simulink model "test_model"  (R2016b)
settings: Solver=VariableStepAuto  StartTime=0.0  StopTime=runtime  RelTol=1e-3
InitFcn:
  | clear mex
  | delete test_model_sfun.mexw64
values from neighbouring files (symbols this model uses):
  delta_T = 4 * [ 0,  0,  2.351e-4 ]    [modelParameters.m]
  Delta_T = cell(1,4)    [modelParameters.m]
  F_D = 1*randn(3,1)    [modelParameters.m]
  g = 9.81    [modelParameters.m]    (also in analyzeIMU_data.m = 9.8; getMomentOfInertia.m = 9.80665)
  Gamma_H = cell(1,4)    [modelParameters.m]
  have_motor_transient = 1    [modelParameters.m]
  height_controlled_o = (((Rm*If        + (((omega0_o * 2 * Rm * Kv * Kq      * Kd + 1)^2) - 1)/(4* Rm*Kv^2*Kq      * Kd))/Vb)*(Pmax - Pmin) + Pmin)    [modelParameters.m]
  i_0 = cell(1,4)    [modelParameters.m]
  If = 0.3836    [modelParameters.m]    (also in thrustDragConstantCalculations.m = [If0; If1; If2; If3]; Kd_error.m = I_0 * sign(rotor_speed_0) + I_1 * rotor_speed_0 + I_2 * roto)
  J = diag([ 0.0130 0.0140 0.0285 ])    [modelParameters.m]    (also in J_calc_bifilar.m = (16*pi^2*L./(m*g.*D.^2))\(t./n).^2)
  J_L = m_L/12*diag([y_L^2+z_L^2,x_L^2+z_L^2,x_L^2+y_L^2])    [modelParameters.m]
  J_r = cell(1,4)    [modelParameters.m]
  Jreq = 4.2012e-05    [modelParameters.m]
  Jxx = 0.0130    (= 0.013)    [modelParameters.m]
  Jyy = 0.0140    (= 0.014)    [modelParameters.m]
  Jzz = 0.0285    [modelParameters.m]
  K_d = cell(1,4)    [modelParameters.m]
  K_E = cell(1,4)    [modelParameters.m]
  K_H = cell(1,4)    [modelParameters.m]
  K_Q = cell(1,4)    [modelParameters.m]
  K_T = cell(1,4)    [modelParameters.m]
  K_V = cell(1,4)    [modelParameters.m]
  Kd = 1.4852e-07    [modelParameters.m]    (also in calcDragConstant.m = ((A'*A)^-1)*A'*b; thrustDragConstantCalculations.m = calcDragConstant(data, Pmin, Pmax, Rm, Kv, Kq, If); Kd_error.m = 1.0317e-07)
  Kh = 3.4574e-04    (= 0.00034574)    [modelParameters.m]
  Ki_mahony = 0.001    [modelParameters.m]
  Kp_mahony = 0.4    [modelParameters.m]
  Kq = 96.3422    [modelParameters.m]    (also in thrustDragConstantCalculations.m; Kd_error.m)
  Kt = 1.2007e-05    [modelParameters.m]    (also in calcThrustConstant.m = ((A'*A)^(-1))*(A'*T); thrustDragConstantCalculations.m = calcThrustConstant(data))
  Kv = 96.3422    [modelParameters.m]    (also in thrustDragConstantCalculations.m; Kd_error.m)
  m = 1.216    [modelParameters.m]
  m_L = 0    [modelParameters.m]
  omega0_o = sqrt((m*g)/(4*Kt))    [modelParameters.m]
  omega1_o = sqrt((m*g)/(4*Kt))    [modelParameters.m]
  omega2_o = sqrt((m*g)/(4*Kt))    [modelParameters.m]
  omega3_o = sqrt((m*g)/(4*Kt))    [modelParameters.m]
  omega_0 = cell(1,4)    [modelParameters.m]
  p0 = 0    [modelParameters.m]
  p_0 = cell(1,4)    [modelParameters.m]
  p_max = cell(1,4)    [modelParameters.m]
  phi0 = 0    [modelParameters.m]
  pitch_o = 0    [modelParameters.m]
  pitchrate_o = 0    [modelParameters.m]
  Pmax = 1    [modelParameters.m]    (also in thrustDragConstantCalculations.m = 200000; Kd_error.m = 200000)
  Pmin = 0    [modelParameters.m]    (also in thrustDragConstantCalculations.m = 100000; Kd_error.m = 100000)
  psi0 = 0    [modelParameters.m]
  q0 = 0    [modelParameters.m]
  Q_D = 0.05*randn(3,1)    [modelParameters.m]
  r0 = 0    [modelParameters.m]
  R_m = cell(1,4)    [modelParameters.m]
  r_oc = [ 0 ; 0 ; 0 ]    [modelParameters.m]
  r_oL = [0; 0; 0]    [modelParameters.m]
  rhx = 0.16    [modelParameters.m]
  rhy = 0.16    [modelParameters.m]
  rhz = 0.03    [modelParameters.m]
  Rm = 0.235    [modelParameters.m]    (also in thrustDragConstantCalculations.m = 0.2308; Kd_error.m = 0.2308)
  roll_o = 0    [modelParameters.m]
  rollrate_o = 0    [modelParameters.m]
  Tc = 0.04    [modelParameters.m]
  theta0 = 0    [modelParameters.m]
  Tq = 0.005    [modelParameters.m]
  u0 = 0    [modelParameters.m]
  v0 = 0    [modelParameters.m]
  Vb = 12.3    [modelParameters.m]    (also in calcDragConstant.m = [data.(6); data.(6); data.(6); data.(6)]; Kd_error.m = data.(6))
  w0 = 0    [modelParameters.m]
  x0 = 0    [modelParameters.m]
  x_controlled_o = 0    [modelParameters.m]
  x_o = 0    [modelParameters.m]
  x_vel_o = 0    [modelParameters.m]
  y0 = 0    [modelParameters.m]
  y_controlled_o = 0    [modelParameters.m]
  y_o = 0    [modelParameters.m]
  y_vel_o = 0    [modelParameters.m]
  yaw_controlled_o = 0    [modelParameters.m]
  yaw_o = 0    [modelParameters.m]
  yawrate_o = 0    [modelParameters.m]
  z0 = 0    [modelParameters.m]
  z_o = 0    [modelParameters.m]
  z_vel_o = 0    [modelParameters.m]
undefined symbols (not defined in the file or in its folder): Gamma_Omega, Gamma_T, Ki, Kp, r_h, slope, start, Ts, X0
libraries: simulink x32, Derivative x26, dsparch4 x6, vrlib x4
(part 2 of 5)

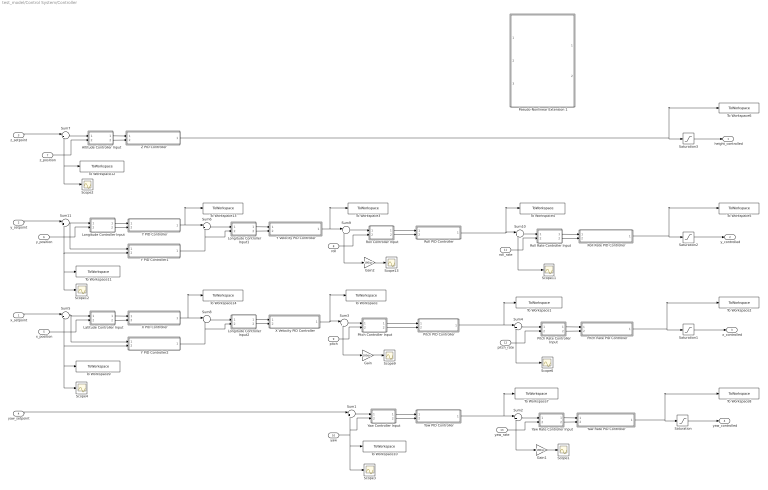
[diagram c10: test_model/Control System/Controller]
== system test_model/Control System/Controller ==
  x_setpoint : Inport
  y_setpoint : Inport  Port=2
  z_setpoint : Inport  Port=3
  yaw_setpoint : Inport  Port=4
  x_position : Inport  Port=5
  y_position : Inport  Port=6
  z_position : Inport  Port=7
  roll : Inport  Port=8
  pitch : Inport  Port=9
  yaw : Inport  Port=10
  roll_rate : Inport  Port=11
  pitch_rate : Inport  Port=12
  yaw_rate : Inport  Port=13
  Altitude Controller Input : Subsystem  Variant=on
  Gain : Gain  Gain=180/pi
  Gain1 : Gain  Gain=180/pi
  Gain2 : Gain  Gain=180/pi
  Latitude Controller Input : Subsystem  Variant=on
  Longitude Controller Input : Subsystem  Variant=on
  Longitude Controller Input1 : Subsystem  Variant=on
  Longitude Controller Input2 : Subsystem  Variant=on
  Pitch Controller Input : Subsystem  Variant=on
  Pitch PID Controller : Subsystem
  Pitch Rate Controller Input : Subsystem  Variant=on
  Pitch Rate PID Controller : Subsystem
  Pseudo-Nonlinear Extension 1 : MATLAB Function  TreatAsAtomicUnit=on
  Roll Controller Input : Subsystem  Variant=on
  Roll PID Controller : Subsystem
  Roll Rate Controller Input : Subsystem  Variant=on
  Roll Rate PID Controller : Subsystem
  Saturation{,1..3} (4 alike) : Saturate  UpperLimit=20000  LowerLimit=-20000
  Scope{1..4,6,9,11..13} (9 alike) : Scope
  Sum{1..11} (11 alike) : Sum  Inputs=|+-
  To Workspace : ToWorkspace  VariableName=pitch_setpoint_model  SaveFormat=Structure With Time  SampleTime=-1
  To Workspace1 : ToWorkspace  VariableName=pitchrate_setpoint_model  SaveFormat=Structure With Time  SampleTime=Tq
  To Workspace10 : ToWorkspace  VariableName=yaw_value_model  SaveFormat=Structure With Time  SampleTime=Tc
  To Workspace11 : ToWorkspace  VariableName=y_position_model  SaveFormat=Structure With Time  SampleTime=Tc
  To Workspace12 : ToWorkspace  VariableName=z_position_model  SaveFormat=Structure With Time  SampleTime=Tc
  To Workspace13 : ToWorkspace  VariableName=y_vel_setpoint_model  SaveFormat=Structure With Time  SampleTime=Tc
  To Workspace14 : ToWorkspace  VariableName=x_vel_setpoint_model  SaveFormat=Structure With Time  SampleTime=Tc
  To Workspace2 : ToWorkspace  VariableName=x_command_model  SaveFormat=Structure With Time  SampleTime=Tq
  To Workspace3 : ToWorkspace  VariableName=roll_setpoint_model  SaveFormat=Structure With Time  SampleTime=Tc
  To Workspace4 : ToWorkspace  VariableName=rollrate_setpoint_model  SaveFormat=Structure With Time  SampleTime=Tq
  To Workspace5 : ToWorkspace  VariableName=y_command_model  SaveFormat=Structure With Time  SampleTime=Tq
  To Workspace6 : ToWorkspace  VariableName=z_command_model  SaveFormat=Structure With Time  SampleTime=Tc
  To Workspace7 : ToWorkspace  VariableName=yawrate_setpoint_model  SaveFormat=Structure With Time  SampleTime=Tc
  To Workspace8 : ToWorkspace  VariableName=yaw_command_model  SaveFormat=Structure With Time  SampleTime=Tq
  To Workspace9 : ToWorkspace  VariableName=x_position_model  SaveFormat=Structure With Time  SampleTime=Tc
  X PID Controller : Subsystem
  X Velocity PID Controller : Subsystem
  Y PID Controller : Subsystem
  Y PID Controller1 : Subsystem
  Y PID Controller2 : Subsystem
  Y Velocity PID Controller : Subsystem
  Yaw Controller Input : Subsystem  Variant=on
  Yaw PID Controller : Subsystem
  Yaw Rate Controller Input : Subsystem  Variant=on
  Yaw Rate PID Controller : Subsystem
  Z PID Controller : Subsystem
  height_controlled : Outport
  y_controlled : Outport  Port=2
  x_controlled : Outport  Port=3
  yaw_controlled : Outport  Port=4
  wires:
  pitch_rate/1 -> Pitch Rate Controller Input/2(pitchrate_model), Scope6/1, Sum4/2
  z_setpoint/1 -> Sum7/1
  x_position/1 -> Sum5/2, Latitude Controller Input/2(x_position_model), Scope4/1, To Workspace9/1, Y PID Controller2/2(x_pos)
  Pitch PID Controller/1(pitchrate_setpoint) -> Sum4/1, To Workspace1/1
  pitch/1 -> Pitch Controller Input/2(pitch_angle_model), Gain/1, Sum3/2
  Gain/1 -> Scope9/1
  Yaw Rate PID Controller/1(yaw_motor_command) -> To Workspace8/1, Saturation/1
  Pitch Rate PID Controller/1(x_motor_command) -> Saturation1/1, To Workspace2/1
  x_setpoint/1 -> Sum5/1
  roll_rate/1 -> Roll Rate Controller Input/2(rollrate_model), Scope11/1, Sum10/2
  Roll PID Controller/1(rollrate_setpoint) -> Sum10/1, To Workspace4/1
  roll/1 -> Roll Controller Input/2(roll_angle_model), Gain2/1, Sum9/2
  Gain2/1 -> Scope13/1
  y_setpoint/1 -> Sum11/1
  yaw/1 -> Yaw Controller Input/2(yaw_angle_model), Sum1/2, Scope3/1, To Workspace10/1
  yaw_setpoint/1 -> Sum1/1
  yaw_rate/1 -> Gain1/1, Yaw Rate Controller Input/2(yawrate_model), Sum2/2
  Gain1/1 -> Scope1/1
  Yaw PID Controller/1(yawrate_setpoint) -> Sum2/1, To Workspace7/1
  z_position/1 -> Altitude Controller Input/2(z_position_model), To Workspace12/1, Scope2/1, Sum7/2
  Sum1/1 -> Yaw Controller Input/1(yaw_error_model)
  Sum2/1 -> Yaw Rate Controller Input/1(yawrate_error_model)
  Sum5/1 -> Latitude Controller Input/1(x_error_model), Y PID Controller2/1(x_error)
  Sum3/1 -> Pitch Controller Input/1(pitch_error_model)
  Sum4/1 -> Pitch Rate Controller Input/1(pitchrate_error_model)
  Sum9/1 -> Roll Controller Input/1(roll_error_model)
  Sum10/1 -> Roll Rate Controller Input/1(rollrate_error_model)
  Sum7/1 -> Altitude Controller Input/1(z_error_model)
  Roll Rate PID Controller/1(y_motor_command) -> To Workspace5/1, Saturation2/1
  Saturation3/1 -> height_controlled/1
  Saturation2/1 -> y_controlled/1
  Saturation1/1 -> x_controlled/1
  Saturation/1 -> yaw_controlled/1
  Longitude Controller Input/2(y_position) -> Y PID Controller/2(y_pos)
  Longitude Controller Input/1(y_error) -> Y PID Controller/1(y_error)
  y_position/1 -> Longitude Controller Input/2(y_position_model), Y PID Controller1/2(y_pos), To Workspace11/1, Scope12/1, Sum11/2
  Latitude Controller Input/1(x_error) -> X PID Controller/1(x_error)
  Latitude Controller Input/2(x_position) -> X PID Controller/2(x_pos)
  Yaw Controller Input/1(yaw_error) -> Yaw PID Controller/1(yaw_error)
  Yaw Controller Input/2(yaw_angle) -> Yaw PID Controller/2(yaw_angle)
  Altitude Controller Input/1(z_error) -> Z PID Controller/1(z_error)
  Altitude Controller Input/2(z_position) -> Z PID Controller/2(z_pos)
  Pitch Controller Input/1(pitch_error) -> Pitch PID Controller/1(pitch_error)
  Pitch Controller Input/2(pitch_angle) -> Pitch PID Controller/2(pitch_angle)
  Yaw Rate Controller Input/1(yawrate_error) -> Yaw Rate PID Controller/1(yawrate_error)
  Yaw Rate Controller Input/2(yawrate) -> Yaw Rate PID Controller/2(yawrate)
  Pitch Rate Controller Input/1(pitchrate_error) -> Pitch Rate PID Controller/1(pitchrate_error)
  Pitch Rate Controller Input/2(pitchrate) -> Pitch Rate PID Controller/2(pitchrate)
  Roll Controller Input/1(roll_error) -> Roll PID Controller/1(roll_error)
  Roll Controller Input/2(roll_angle) -> Roll PID Controller/2(roll_angle)
  Roll Rate Controller Input/1(rollrate_error) -> Roll Rate PID Controller/1(rollrate_error)
  Roll Rate Controller Input/2(rollrate) -> Roll Rate PID Controller/2(rollrate)
  Sum11/1 -> Longitude Controller Input/1(y_error_model), Y PID Controller1/1(y_error)
  Y PID Controller/1(roll_setpoint) -> To Workspace13/1, Sum6/1
  Y PID Controller1/1(y_vel_setpoint) -> Longitude Controller Input1/2(y_vel_model), Sum6/2
  Sum6/1 -> Longitude Controller Input1/1(y_vel_error_model)
  Longitude Controller Input1/1(y_vel_error) -> Y Velocity PID Controller/1(y_error)
  Longitude Controller Input1/2(y_vel) -> Y Velocity PID Controller/2(y_pos)
  X PID Controller/1(pitch_setpoint) -> To Workspace14/1, Sum8/1
  Y PID Controller2/1(x_vel_setpoint) -> Longitude Controller Input2/2(x_vel_model), Sum8/2
  Sum8/1 -> Longitude Controller Input2/1(x_vel_error_model)
  Longitude Controller Input2/1(x_vel_error) -> X Velocity PID Controller/1(x_vel_error)
  Longitude Controller Input2/2(x_vel) -> X Velocity PID Controller/2(x_vel)
  Z PID Controller/1(z_motor_command) -> To Workspace6/1, Saturation3/1
  Y Velocity PID Controller/1(roll_setpoint) -> To Workspace3/1, Sum9/1
  X Velocity PID Controller/1(pitch_setpoint) -> To Workspace/1, Sum3/1

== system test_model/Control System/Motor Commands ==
  note: 1) Add Subsystem or Model blocks as valid variant choices. 2) You cannot connect blocks at this level. At simulation, connectivity is automatically determined, based on the active variant and port name matching.
  z_command_model : Inport
  Feedback : Subsystem  VariantControl=logAnalysisToggle==0
  Motor Command : Subsystem  VariantControl=logAnalysisToggle==1
  z_command : Outport

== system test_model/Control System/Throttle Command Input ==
  note: 1) Add Subsystem or Model blocks as valid variant choices. 2) You cannot connect blocks at this level. At simulation, connectivity is automatically determined, based on the active variant and port name matching.
  Auto Takeoff : Subsystem  VariantControl=logAnalysisToggle==1
  height_controlled_o : Subsystem  VariantControl=logAnalysisToggle==0
  z_command : Outport

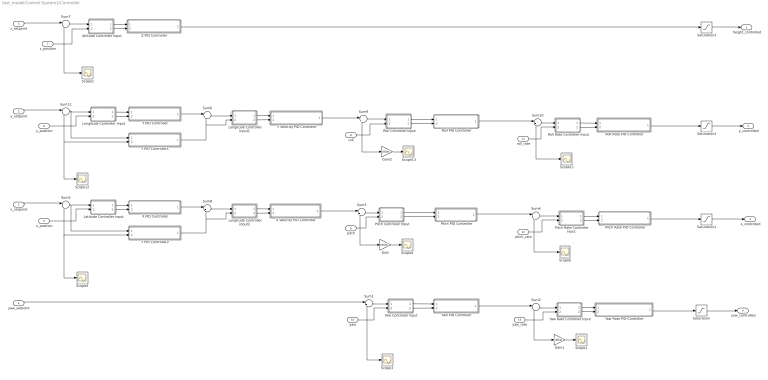
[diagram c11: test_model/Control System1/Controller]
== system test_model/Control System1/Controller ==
  x_setpoint : Inport
  y_setpoint : Inport  Port=2
  z_setpoint : Inport  Port=3
  yaw_setpoint : Inport  Port=4
  x_position : Inport  Port=5
  y_position : Inport  Port=6
  z_position : Inport  Port=7
  roll : Inport  Port=8
  pitch : Inport  Port=9
  yaw : Inport  Port=10
  roll_rate : Inport  Port=11
  pitch_rate : Inport  Port=12
  yaw_rate : Inport  Port=13
  Altitude Controller Input : Subsystem  Variant=on
  Gain : Gain  Gain=180/pi
  Gain1 : Gain  Gain=180/pi
  Gain2 : Gain  Gain=180/pi
  Latitude Controller Input : Subsystem  Variant=on
  Longitude Controller Input : Subsystem  Variant=on
  Longitude Controller Input1 : Subsystem  Variant=on
  Longitude Controller Input2 : Subsystem  Variant=on
  Pitch Controller Input : Subsystem  Variant=on
  Pitch PID Controller : Subsystem
  Pitch Rate Controller Input : Subsystem  Variant=on
  Pitch Rate PID Controller : Subsystem
  Roll Controller Input : Subsystem  Variant=on
  Roll PID Controller : Subsystem
  Roll Rate Controller Input : Subsystem  Variant=on
  Roll Rate PID Controller : Subsystem
  Saturation{,1..3} (4 alike) : Saturate  UpperLimit=20000  LowerLimit=-20000
  Scope{1..4,6,9,11..13} (9 alike) : Scope
  Sum{1..11} (11 alike) : Sum  Inputs=|+-
  X PID Controller : Subsystem
  X Velocity PID Controller : Subsystem
  Y PID Controller : Subsystem
  Y PID Controller1 : Subsystem
  Y PID Controller2 : Subsystem
  Y Velocity PID Controller : Subsystem
  Yaw Controller Input : Subsystem  Variant=on
  Yaw PID Controller : Subsystem
  Yaw Rate Controller Input : Subsystem  Variant=on
  Yaw Rate PID Controller : Subsystem
  Z PID Controller : Subsystem
  height_controlled : Outport
  y_controlled : Outport  Port=2
  x_controlled : Outport  Port=3
  yaw_controlled : Outport  Port=4
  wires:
  pitch_rate/1 -> Pitch Rate Controller Input/2(pitchrate_model), Scope6/1, Sum4/2
  z_setpoint/1 -> Sum7/1
  x_position/1 -> Sum5/2, Latitude Controller Input/2(x_position_model), Scope4/1, Y PID Controller2/2(x_pos)
  Pitch PID Controller/1(pitchrate_setpoint) -> Sum4/1
  pitch/1 -> Pitch Controller Input/2(pitch_angle_model), Gain/1, Sum3/2
  Gain/1 -> Scope9/1
  Yaw Rate PID Controller/1(yaw_motor_command) -> Saturation/1
  Pitch Rate PID Controller/1(x_motor_command) -> Saturation1/1
  x_setpoint/1 -> Sum5/1
  roll_rate/1 -> Roll Rate Controller Input/2(rollrate_model), Scope11/1, Sum10/2
  Roll PID Controller/1(rollrate_setpoint) -> Sum10/1
  roll/1 -> Roll Controller Input/2(roll_angle_model), Gain2/1, Sum9/2
  Gain2/1 -> Scope13/1
  y_setpoint/1 -> Sum11/1
  yaw/1 -> Yaw Controller Input/2(yaw_angle_model), Scope3/1, Sum1/2
  yaw_setpoint/1 -> Sum1/1
  yaw_rate/1 -> Gain1/1, Yaw Rate Controller Input/2(yawrate_model), Sum2/2
  Gain1/1 -> Scope1/1
  Yaw PID Controller/1(yawrate_setpoint) -> Sum2/1
  z_position/1 -> Altitude Controller Input/2(z_position_model), Scope2/1, Sum7/2
  Sum1/1 -> Yaw Controller Input/1(yaw_error_model)
  Sum2/1 -> Yaw Rate Controller Input/1(yawrate_error_model)
  Sum5/1 -> Latitude Controller Input/1(x_error_model), Y PID Controller2/1(x_error)
  Sum3/1 -> Pitch Controller Input/1(pitch_error_model)
  Sum4/1 -> Pitch Rate Controller Input/1(pitchrate_error_model)
  Sum9/1 -> Roll Controller Input/1(roll_error_model)
  Sum10/1 -> Roll Rate Controller Input/1(rollrate_error_model)
  Sum7/1 -> Altitude Controller Input/1(z_error_model)
  Roll Rate PID Controller/1(y_motor_command) -> Saturation2/1
  Saturation3/1 -> height_controlled/1
  Saturation2/1 -> y_controlled/1
  Saturation1/1 -> x_controlled/1
  Saturation/1 -> yaw_controlled/1
  Longitude Controller Input/2(y_position) -> Y PID Controller/2(y_pos)
  Longitude Controller Input/1(y_error) -> Y PID Controller/1(y_error)
  y_position/1 -> Longitude Controller Input/2(y_position_model), Y PID Controller1/2(y_pos), Scope12/1, Sum11/2
  Latitude Controller Input/1(x_error) -> X PID Controller/1(x_error)
  Latitude Controller Input/2(x_position) -> X PID Controller/2(x_pos)
  Yaw Controller Input/1(yaw_error) -> Yaw PID Controller/1(yaw_error)
  Yaw Controller Input/2(yaw_angle) -> Yaw PID Controller/2(yaw_angle)
  Altitude Controller Input/1(z_error) -> Z PID Controller/1(z_error)
  Altitude Controller Input/2(z_position) -> Z PID Controller/2(z_pos)
  Pitch Controller Input/1(pitch_error) -> Pitch PID Controller/1(pitch_error)
  Pitch Controller Input/2(pitch_angle) -> Pitch PID Controller/2(pitch_angle)
  Yaw Rate Controller Input/1(yawrate_error) -> Yaw Rate PID Controller/1(yawrate_error)
  Yaw Rate Controller Input/2(yawrate) -> Yaw Rate PID Controller/2(yawrate)
  Pitch Rate Controller Input/1(pitchrate_error) -> Pitch Rate PID Controller/1(pitchrate_error)
  Pitch Rate Controller Input/2(pitchrate) -> Pitch Rate PID Controller/2(pitchrate)
  Roll Controller Input/1(roll_error) -> Roll PID Controller/1(roll_error)
  Roll Controller Input/2(roll_angle) -> Roll PID Controller/2(roll_angle)
  Roll Rate Controller Input/1(rollrate_error) -> Roll Rate PID Controller/1(rollrate_error)
  Roll Rate Controller Input/2(rollrate) -> Roll Rate PID Controller/2(rollrate)
  Sum11/1 -> Longitude Controller Input/1(y_error_model), Y PID Controller1/1(y_error)
  Y PID Controller/1(roll_setpoint) -> Sum6/1
  Y PID Controller1/1(y_vel_setpoint) -> Longitude Controller Input1/2(y_vel_model), Sum6/2
  Sum6/1 -> Longitude Controller Input1/1(y_vel_error_model)
  Longitude Controller Input1/1(y_vel_error) -> Y Velocity PID Controller/1(y_error)
  Longitude Controller Input1/2(y_vel) -> Y Velocity PID Controller/2(y_pos)
  Y Velocity PID Controller/1(roll_setpoint) -> Sum9/1
  X PID Controller/1(pitch_setpoint) -> Sum8/1
  Y PID Controller2/1(x_vel_setpoint) -> Longitude Controller Input2/2(x_vel_model), Sum8/2
  Sum8/1 -> Longitude Controller Input2/1(x_vel_error_model)
  Longitude Controller Input2/1(x_vel_error) -> X Velocity PID Controller/1(x_vel_error)
  Longitude Controller Input2/2(x_vel) -> X Velocity PID Controller/2(x_vel)
  X Velocity PID Controller/1(pitch_setpoint) -> Sum3/1
  Z PID Controller/1(z_motor_command) -> Saturation3/1

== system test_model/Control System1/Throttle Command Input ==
  note: 1) Add Subsystem or Model blocks as valid variant choices. 2) You cannot connect blocks at this level. At simulation, connectivity is automatically determined, based on the active variant and port name matching.
  Auto Takeoff : Subsystem  VariantControl=logAnalysisToggle==1
  height_controlled_o : Subsystem  VariantControl=logAnalysisToggle==0
  z_command : Outport

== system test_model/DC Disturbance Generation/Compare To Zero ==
  u : Inport
  Compare : RelationalOperator  Operator=~=  OutDataTypeStr=fixdt(0, 8)
  Constant : Constant  DisableCoverage=on  Value=0  OutDataTypeStr=Inherit: Inherit via back propagation  PreserveConstantTs=on
  y : Outport
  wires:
  Constant/1 -> Compare/2
  u/1 -> Compare/1
  Compare/1 -> y/1

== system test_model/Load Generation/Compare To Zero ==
  u : Inport
  Compare : RelationalOperator  Operator=~=  OutDataTypeStr=fixdt(0, 8)
  Constant : Constant  DisableCoverage=on  Value=0  OutDataTypeStr=Inherit: Inherit via back propagation  PreserveConstantTs=on
  y : Outport
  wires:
  Constant/1 -> Compare/2
  u/1 -> Compare/1
  Compare/1 -> y/1

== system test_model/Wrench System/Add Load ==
  m_0 : Inport
  J_0 : Inport  Port=2
  r_oc_0 : Inport  Port=3
  m_l : Inport  Port=4
  J_l : Inport  Port=5
  r_ol : Inport  Port=6
  Add Load to Quadrotor : MATLAB Function  TreatAsAtomicUnit=on
  m : Outport
  J : Outport  Port=2
  r_oc : Outport  Port=3
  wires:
  r_ol/1 -> Add Load to Quadrotor/6(r_ol)
  Add Load to Quadrotor/3(r_oc) -> r_oc/1
  J_l/1 -> Add Load to Quadrotor/5(J_l)
  m_l/1 -> Add Load to Quadrotor/4(m_l)
  Add Load to Quadrotor/2(J) -> J/1
  r_oc_0/1 -> Add Load to Quadrotor/3(r_oc_0)
  J_0/1 -> Add Load to Quadrotor/2(J_0)
  Add Load to Quadrotor/1(m) -> m/1
  m_0/1 -> Add Load to Quadrotor/1(m_0)

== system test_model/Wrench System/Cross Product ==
  note: Cross product of two 3x1 vectors a=[a1 a2 a3], b=[b1 b2 b3]: y = a x b = (a2b3 - a3b2)i + (a3b1 - a1b3)j + (a1b2 - a2b1)k
  a : Inport
  b : Inport  Port=2
  Add3 : Sum  Inputs=+-
  Demux2 : Demux  Outputs=2
  Element product : Product
  a elements : Selector  InputPortWidth=3  IndexOptions=Index vector (dialog)  Indices=[2 3 1 3 1 2]  OutputSizes=1
  b elements : Selector  InputPortWidth=3  IndexOptions=Index vector (dialog)  Indices=[3 1 2 2 3 1]  OutputSizes=1
  y : Outport
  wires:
  Add3/1 -> y/1
  Demux2/2 -> Add3/2
  Demux2/1 -> Add3/1
  Element product/1 -> Demux2/1
  a/1 -> a elements/1
  b/1 -> b elements/1
  b elements/1 -> Element product/2
  a elements/1 -> Element product/1

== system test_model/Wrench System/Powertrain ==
  P : Inport
  Lambda : Inport  Port=2
  8 Inch Rotor System : Subsystem
  Battery : Subsystem
  ESC-BLDC Motor System : Subsystem
  W_r : Outport
  M : Outport  Port=2
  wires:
  8 Inch Rotor System/1(W_r) -> W_r/1
  Lambda/1 -> 8 Inch Rotor System/2(Lambda)
  P/1 -> ESC-BLDC Motor System/1(P)
  Battery/1(V) -> ESC-BLDC Motor System/2(V_b)
  ESC-BLDC Motor System/1(M) -> 8 Inch Rotor System/1(M), M/1

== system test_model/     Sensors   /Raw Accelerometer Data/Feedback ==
  raw_accel_model : Inport
  raw_accel : Outport
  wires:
  raw_accel_model/1 -> raw_accel/1

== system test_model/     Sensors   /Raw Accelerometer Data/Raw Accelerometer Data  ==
  From Workspace5 : FromWorkspace  VariableName=raw_accel_data  SampleTime=Tq
  raw_accel : Outport
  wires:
  From Workspace5/1 -> raw_accel/1

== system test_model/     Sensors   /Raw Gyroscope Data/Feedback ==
  raw_gyro_model : Inport
  raw_gyro : Outport
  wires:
  raw_gyro_model/1 -> raw_gyro/1

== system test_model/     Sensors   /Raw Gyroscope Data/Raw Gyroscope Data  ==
  From Workspace5 : FromWorkspace  VariableName=raw_gyro_data  SampleTime=Tq
  raw_gyro : Outport
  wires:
  From Workspace5/1 -> raw_gyro/1

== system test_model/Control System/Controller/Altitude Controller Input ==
  note: 1) Add Subsystem or Model blocks as valid variant choices. 2) You cannot connect blocks at this level. At simulation, connectivity is automatically determined, based on the active variant and port name matching.
  z_error_model : Inport
  z_position_model : Inport  Port=2
  Feedback : Subsystem  VariantControl=logAnalysisToggle==0
  z error : Subsystem  VariantControl=logAnalysisToggle==1
  z_error : Outport
  z_position : Outport  Port=2

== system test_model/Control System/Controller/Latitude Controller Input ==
  note: 1) Add Subsystem or Model blocks as valid variant choices. 2) You cannot connect blocks at this level. At simulation, connectivity is automatically determined, based on the active variant and port name matching.
  x_error_model : Inport
  x_position_model : Inport  Port=2
  Feedback : Subsystem  VariantControl=logAnalysisToggle==0
  log : Subsystem  VariantControl=logAnalysisToggle==1
  x_error : Outport
  x_position : Outport  Port=2

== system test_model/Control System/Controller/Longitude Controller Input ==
  note: 1) Add Subsystem or Model blocks as valid variant choices. 2) You cannot connect blocks at this level. At simulation, connectivity is automatically determined, based on the active variant and port name matching.
  y_error_model : Inport
  y_position_model : Inport  Port=2
  Feedback : Subsystem  VariantControl=logAnalysisToggle==0
  y error : Subsystem  VariantControl=logAnalysisToggle==1
  y_error : Outport
  y_position : Outport  Port=2

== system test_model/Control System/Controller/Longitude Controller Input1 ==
  note: 1) Add Subsystem or Model blocks as valid variant choices. 2) You cannot connect blocks at this level. At simulation, connectivity is automatically determined, based on the active variant and port name matching.
  y_vel_error_model : Inport
  y_vel_model : Inport  Port=2
  Feedback : Subsystem  VariantControl=logAnalysisToggle==0
  y error : Subsystem  VariantControl=logAnalysisToggle==1
  y_vel_error : Outport
  y_vel : Outport  Port=2

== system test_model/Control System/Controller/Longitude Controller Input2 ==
  note: 1) Add Subsystem or Model blocks as valid variant choices. 2) You cannot connect blocks at this level. At simulation, connectivity is automatically determined, based on the active variant and port name matching.
  x_vel_error_model : Inport
  x_vel_model : Inport  Port=2
  Feedback : Subsystem  VariantControl=logAnalysisToggle==0
  y error : Subsystem  VariantControl=logAnalysisToggle==1
  x_vel_error : Outport
  x_vel : Outport  Port=2

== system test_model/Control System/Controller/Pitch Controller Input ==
  note: 1) Add Subsystem or Model blocks as valid variant choices. 2) You cannot connect blocks at this level. At simulation, connectivity is automatically determined, based on the active variant and port name matching.
  pitch_error_model : Inport
  pitch_angle_model : Inport  Port=2
  Feedback : Subsystem  VariantControl=logAnalysisToggle==0
  pitch error : Subsystem  VariantControl=logAnalysisToggle==1
  pitch_error : Outport
  pitch_angle : Outport  Port=2

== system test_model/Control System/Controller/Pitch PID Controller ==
  pitch_error : Inport
  pitch_angle : Inport  Port=2
  Add : Sum  Inputs=+-
  Discrete D Controller : Derivative/Discrete D Controller  Kd=Kd  a=a
  Discrete PI Controller : simulink/Continuous/PID Controller  Controller=PI  TimeDomain=Discrete-time  SampleTime=Ts  IntegratorMethod=Forward Euler  FilterMethod=Forward Euler  Form=Parallel  UseFilter=on  ControllerParametersSource=internal  P=Kp  I=Ki  D=0  N=100  InitialConditionSource=internal  InitialConditionForIntegrator=0  InitialConditionForFilter=0  ExternalReset=none  LimitOutput=off  UpperSaturationLimit=inf  LowerSaturationLimit=-inf  LinearizeAsGain=off  AntiWindupMode=none  Kb=1  TrackingMode=off  Kt=1  PParamMin=[]  PParamMax=[]  IParamMin=[]  IParamMax=[]  DParamMin=[]  DParamMax=[]  NParamMin=[]  NParamMax=[]  KbParamMin=[]  KbParamMax=[]  KtParamMin=[]  KtParamMax=[]  POutMin=[]  POutMax=[]  IOutMin=[]  IOutMax=[]  DOutMin=[]  DOutMax=[]  NOutMin=[]  NOutMax=[]  KbOutMin=[]  KbOutMax=[]  KtOutMin=[]  KtOutMax=[]  IntegratorOutMin=[]  IntegratorOutMax=[]  FilterOutMin=[]  FilterOutMax=[]  SumOutMin=[]  SumOutMax=[]  SumI1OutMin=[]  SumI1OutMax=[]  SumI2OutMin=[]  SumI2OutMax=[]  SumI3OutMin=[]  SumI3OutMax=[]  SumDOutMin=[]  SumDOutMax=[]  SaturationOutMin=[]  SaturationOutMax=[]  IntegratorContinuousStateAttributes=''  IntegratorStateMustResolveToSignalObject=off  IntegratorRTWStateStorageClass=Auto  FilterContinuousStateAttributes=''  FilterStateMustResolveToSignalObject=off  FilterRTWStateStorageClass=Auto  DifferentiatorICPrevScaledInput=0  DifferentiatorOutMin=[]  DifferentiatorOutMax=[]
  pitchrate_setpoint : Outport
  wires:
  pitch_angle/1 -> Discrete D Controller/1
  pitch_error/1 -> Discrete PI Controller/1
  Discrete PI Controller/1 -> Add/1
  Discrete D Controller/1 -> Add/2
  Add/1 -> pitchrate_setpoint/1

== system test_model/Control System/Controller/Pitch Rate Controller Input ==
  note: 1) Add Subsystem or Model blocks as valid variant choices. 2) You cannot connect blocks at this level. At simulation, connectivity is automatically determined, based on the active variant and port name matching.
  pitchrate_error_model : Inport
  pitchrate_model : Inport  Port=2
  Feedback : Subsystem  VariantControl=logAnalysisToggle==0
  pitchrate error : Subsystem  VariantControl=logAnalysisToggle==1
  pitchrate_error : Outport
  pitchrate : Outport  Port=2

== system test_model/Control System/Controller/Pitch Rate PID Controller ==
  pitchrate_error : Inport
  pitchrate : Inport  Port=2
  Add : Sum  Inputs=+-
  Discrete D Controller : Derivative/Discrete D Controller  Kd=Kd  a=a
  Discrete PI Controller : simulink/Continuous/PID Controller  Controller=PI  TimeDomain=Discrete-time  SampleTime=Ts  IntegratorMethod=Forward Euler  FilterMethod=Forward Euler  Form=Parallel  UseFilter=on  ControllerParametersSource=internal  P=Kp  I=Ki  D=0  N=100  InitialConditionSource=internal  InitialConditionForIntegrator=0  InitialConditionForFilter=0  ExternalReset=none  LimitOutput=off  UpperSaturationLimit=inf  LowerSaturationLimit=-inf  LinearizeAsGain=off  AntiWindupMode=none  Kb=1  TrackingMode=off  Kt=1  PParamMin=[]  PParamMax=[]  IParamMin=[]  IParamMax=[]  DParamMin=[]  DParamMax=[]  NParamMin=[]  NParamMax=[]  KbParamMin=[]  KbParamMax=[]  KtParamMin=[]  KtParamMax=[]  POutMin=[]  POutMax=[]  IOutMin=[]  IOutMax=[]  DOutMin=[]  DOutMax=[]  NOutMin=[]  NOutMax=[]  KbOutMin=[]  KbOutMax=[]  KtOutMin=[]  KtOutMax=[]  IntegratorOutMin=[]  IntegratorOutMax=[]  FilterOutMin=[]  FilterOutMax=[]  SumOutMin=[]  SumOutMax=[]  SumI1OutMin=[]  SumI1OutMax=[]  SumI2OutMin=[]  SumI2OutMax=[]  SumI3OutMin=[]  SumI3OutMax=[]  SumDOutMin=[]  SumDOutMax=[]  SaturationOutMin=[]  SaturationOutMax=[]  IntegratorContinuousStateAttributes=''  IntegratorStateMustResolveToSignalObject=off  IntegratorRTWStateStorageClass=Auto  FilterContinuousStateAttributes=''  FilterStateMustResolveToSignalObject=off  FilterRTWStateStorageClass=Auto  DifferentiatorICPrevScaledInput=0  DifferentiatorOutMin=[]  DifferentiatorOutMax=[]
  x_motor_command : Outport
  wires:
  pitchrate/1 -> Discrete D Controller/1
  pitchrate_error/1 -> Discrete PI Controller/1
  Discrete PI Controller/1 -> Add/1
  Discrete D Controller/1 -> Add/2
  Add/1 -> x_motor_command/1

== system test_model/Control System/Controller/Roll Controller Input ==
  note: 1) Add Subsystem or Model blocks as valid variant choices. 2) You cannot connect blocks at this level. At simulation, connectivity is automatically determined, based on the active variant and port name matching.
  roll_error_model : Inport
  roll_angle_model : Inport  Port=2
  Feedback : Subsystem  VariantControl=logAnalysisToggle==0
  roll error : Subsystem  VariantControl=logAnalysisToggle==1
  roll_error : Outport
  roll_angle : Outport  Port=2

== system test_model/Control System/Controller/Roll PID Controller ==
  roll_error : Inport
  roll_angle : Inport  Port=2
  Add : Sum  Inputs=+-
  Discrete D Controller : Derivative/Discrete D Controller  Kd=Kd  a=a
  Discrete PI Controller : simulink/Continuous/PID Controller  Controller=PI  TimeDomain=Discrete-time  SampleTime=Ts  IntegratorMethod=Forward Euler  FilterMethod=Forward Euler  Form=Parallel  UseFilter=on  ControllerParametersSource=internal  P=Kp  I=Ki  D=0  N=100  InitialConditionSource=internal  InitialConditionForIntegrator=0  InitialConditionForFilter=0  ExternalReset=none  LimitOutput=off  UpperSaturationLimit=inf  LowerSaturationLimit=-inf  LinearizeAsGain=off  AntiWindupMode=none  Kb=1  TrackingMode=off  Kt=1  PParamMin=[]  PParamMax=[]  IParamMin=[]  IParamMax=[]  DParamMin=[]  DParamMax=[]  NParamMin=[]  NParamMax=[]  KbParamMin=[]  KbParamMax=[]  KtParamMin=[]  KtParamMax=[]  POutMin=[]  POutMax=[]  IOutMin=[]  IOutMax=[]  DOutMin=[]  DOutMax=[]  NOutMin=[]  NOutMax=[]  KbOutMin=[]  KbOutMax=[]  KtOutMin=[]  KtOutMax=[]  IntegratorOutMin=[]  IntegratorOutMax=[]  FilterOutMin=[]  FilterOutMax=[]  SumOutMin=[]  SumOutMax=[]  SumI1OutMin=[]  SumI1OutMax=[]  SumI2OutMin=[]  SumI2OutMax=[]  SumI3OutMin=[]  SumI3OutMax=[]  SumDOutMin=[]  SumDOutMax=[]  SaturationOutMin=[]  SaturationOutMax=[]  IntegratorContinuousStateAttributes=''  IntegratorStateMustResolveToSignalObject=off  IntegratorRTWStateStorageClass=Auto  FilterContinuousStateAttributes=''  FilterStateMustResolveToSignalObject=off  FilterRTWStateStorageClass=Auto  DifferentiatorICPrevScaledInput=0  DifferentiatorOutMin=[]  DifferentiatorOutMax=[]
  rollrate_setpoint : Outport
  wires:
  roll_angle/1 -> Discrete D Controller/1
  roll_error/1 -> Discrete PI Controller/1
  Discrete PI Controller/1 -> Add/1
  Discrete D Controller/1 -> Add/2
  Add/1 -> rollrate_setpoint/1

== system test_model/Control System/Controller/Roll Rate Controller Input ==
  note: 1) Add Subsystem or Model blocks as valid variant choices. 2) You cannot connect blocks at this level. At simulation, connectivity is automatically determined, based on the active variant and port name matching.
  rollrate_error_model : Inport
  rollrate_model : Inport  Port=2
  Feedback : Subsystem  VariantControl=logAnalysisToggle==0
  rollrate error : Subsystem  VariantControl=logAnalysisToggle==1
  rollrate_error : Outport
  rollrate : Outport  Port=2

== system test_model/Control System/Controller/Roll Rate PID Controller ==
  rollrate_error : Inport
  rollrate : Inport  Port=2
  Add : Sum  Inputs=+-
  Discrete D Controller : Derivative/Discrete D Controller  Kd=Kd  a=a
  Discrete PI Controller : simulink/Continuous/PID Controller  Controller=PI  TimeDomain=Discrete-time  SampleTime=Ts  IntegratorMethod=Forward Euler  FilterMethod=Forward Euler  Form=Parallel  UseFilter=on  ControllerParametersSource=internal  P=Kp  I=Ki  D=0  N=100  InitialConditionSource=internal  InitialConditionForIntegrator=0  InitialConditionForFilter=0  ExternalReset=none  LimitOutput=off  UpperSaturationLimit=inf  LowerSaturationLimit=-inf  LinearizeAsGain=off  AntiWindupMode=none  Kb=1  TrackingMode=off  Kt=1  PParamMin=[]  PParamMax=[]  IParamMin=[]  IParamMax=[]  DParamMin=[]  DParamMax=[]  NParamMin=[]  NParamMax=[]  KbParamMin=[]  KbParamMax=[]  KtParamMin=[]  KtParamMax=[]  POutMin=[]  POutMax=[]  IOutMin=[]  IOutMax=[]  DOutMin=[]  DOutMax=[]  NOutMin=[]  NOutMax=[]  KbOutMin=[]  KbOutMax=[]  KtOutMin=[]  KtOutMax=[]  IntegratorOutMin=[]  IntegratorOutMax=[]  FilterOutMin=[]  FilterOutMax=[]  SumOutMin=[]  SumOutMax=[]  SumI1OutMin=[]  SumI1OutMax=[]  SumI2OutMin=[]  SumI2OutMax=[]  SumI3OutMin=[]  SumI3OutMax=[]  SumDOutMin=[]  SumDOutMax=[]  SaturationOutMin=[]  SaturationOutMax=[]  IntegratorContinuousStateAttributes=''  IntegratorStateMustResolveToSignalObject=off  IntegratorRTWStateStorageClass=Auto  FilterContinuousStateAttributes=''  FilterStateMustResolveToSignalObject=off  FilterRTWStateStorageClass=Auto  DifferentiatorICPrevScaledInput=0  DifferentiatorOutMin=[]  DifferentiatorOutMax=[]
  y_motor_command : Outport
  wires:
  rollrate/1 -> Discrete D Controller/1
  rollrate_error/1 -> Discrete PI Controller/1
  Discrete PI Controller/1 -> Add/1
  Discrete D Controller/1 -> Add/2
  Add/1 -> y_motor_command/1

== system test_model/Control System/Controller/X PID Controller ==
  x_error : Inport
  x_pos : Inport  Port=2
  Add : Sum  Inputs=+-
  Discrete D Controller : Derivative/Discrete D Controller  Kd=Kd  a=a
  Discrete PI Controller : simulink/Continuous/PID Controller  Controller=PI  TimeDomain=Discrete-time  SampleTime=Ts  IntegratorMethod=Forward Euler  FilterMethod=Forward Euler  Form=Parallel  UseFilter=on  ControllerParametersSource=internal  P=Kp  I=Ki  D=0  N=100  InitialConditionSource=internal  InitialConditionForIntegrator=0  InitialConditionForFilter=0  ExternalReset=none  LimitOutput=off  UpperSaturationLimit=inf  LowerSaturationLimit=-inf  LinearizeAsGain=off  AntiWindupMode=none  Kb=1  TrackingMode=off  Kt=1  PParamMin=[]  PParamMax=[]  IParamMin=[]  IParamMax=[]  DParamMin=[]  DParamMax=[]  NParamMin=[]  NParamMax=[]  KbParamMin=[]  KbParamMax=[]  KtParamMin=[]  KtParamMax=[]  POutMin=[]  POutMax=[]  IOutMin=[]  IOutMax=[]  DOutMin=[]  DOutMax=[]  NOutMin=[]  NOutMax=[]  KbOutMin=[]  KbOutMax=[]  KtOutMin=[]  KtOutMax=[]  IntegratorOutMin=[]  IntegratorOutMax=[]  FilterOutMin=[]  FilterOutMax=[]  SumOutMin=[]  SumOutMax=[]  SumI1OutMin=[]  SumI1OutMax=[]  SumI2OutMin=[]  SumI2OutMax=[]  SumI3OutMin=[]  SumI3OutMax=[]  SumDOutMin=[]  SumDOutMax=[]  SaturationOutMin=[]  SaturationOutMax=[]  IntegratorContinuousStateAttributes=''  IntegratorStateMustResolveToSignalObject=off  IntegratorRTWStateStorageClass=Auto  FilterContinuousStateAttributes=''  FilterStateMustResolveToSignalObject=off  FilterRTWStateStorageClass=Auto  DifferentiatorICPrevScaledInput=0  DifferentiatorOutMin=[]  DifferentiatorOutMax=[]
  pitch_setpoint : Outport
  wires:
  x_pos/1 -> Discrete D Controller/1
  x_error/1 -> Discrete PI Controller/1
  Discrete PI Controller/1 -> Add/1
  Discrete D Controller/1 -> Add/2
  Add/1 -> pitch_setpoint/1

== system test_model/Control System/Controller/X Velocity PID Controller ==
  x_vel_error : Inport
  x_vel : Inport  Port=2
  Add : Sum  Inputs=+-
  Discrete D Controller : Derivative/Discrete D Controller  Kd=Kd  a=a
  Discrete PI Controller : simulink/Continuous/PID Controller  Controller=PI  TimeDomain=Discrete-time  SampleTime=Ts  IntegratorMethod=Forward Euler  FilterMethod=Forward Euler  Form=Parallel  UseFilter=on  ControllerParametersSource=internal  P=Kp  I=Ki  D=0  N=100  InitialConditionSource=internal  InitialConditionForIntegrator=0  InitialConditionForFilter=0  ExternalReset=none  LimitOutput=off  UpperSaturationLimit=inf  LowerSaturationLimit=-inf  LinearizeAsGain=off  AntiWindupMode=none  Kb=1  TrackingMode=off  Kt=1  PParamMin=[]  PParamMax=[]  IParamMin=[]  IParamMax=[]  DParamMin=[]  DParamMax=[]  NParamMin=[]  NParamMax=[]  KbParamMin=[]  KbParamMax=[]  KtParamMin=[]  KtParamMax=[]  POutMin=[]  POutMax=[]  IOutMin=[]  IOutMax=[]  DOutMin=[]  DOutMax=[]  NOutMin=[]  NOutMax=[]  KbOutMin=[]  KbOutMax=[]  KtOutMin=[]  KtOutMax=[]  IntegratorOutMin=[]  IntegratorOutMax=[]  FilterOutMin=[]  FilterOutMax=[]  SumOutMin=[]  SumOutMax=[]  SumI1OutMin=[]  SumI1OutMax=[]  SumI2OutMin=[]  SumI2OutMax=[]  SumI3OutMin=[]  SumI3OutMax=[]  SumDOutMin=[]  SumDOutMax=[]  SaturationOutMin=[]  SaturationOutMax=[]  IntegratorContinuousStateAttributes=''  IntegratorStateMustResolveToSignalObject=off  IntegratorRTWStateStorageClass=Auto  FilterContinuousStateAttributes=''  FilterStateMustResolveToSignalObject=off  FilterRTWStateStorageClass=Auto  DifferentiatorICPrevScaledInput=0  DifferentiatorOutMin=[]  DifferentiatorOutMax=[]
  pitch_setpoint : Outport
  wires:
  x_vel/1 -> Discrete D Controller/1
  x_vel_error/1 -> Discrete PI Controller/1
  Discrete PI Controller/1 -> Add/1
  Discrete D Controller/1 -> Add/2
  Add/1 -> pitch_setpoint/1

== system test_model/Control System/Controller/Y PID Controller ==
  y_error : Inport
  y_pos : Inport  Port=2
  Add : Sum  Inputs=+-
  Discrete D Controller : Derivative/Discrete D Controller  Kd=Kd  a=a
  Discrete PI Controller : simulink/Continuous/PID Controller  Controller=PI  TimeDomain=Discrete-time  SampleTime=Ts  IntegratorMethod=Forward Euler  FilterMethod=Forward Euler  Form=Parallel  UseFilter=on  ControllerParametersSource=internal  P=Kp  I=Ki  D=0  N=100  InitialConditionSource=internal  InitialConditionForIntegrator=0  InitialConditionForFilter=0  ExternalReset=none  LimitOutput=off  UpperSaturationLimit=inf  LowerSaturationLimit=-inf  LinearizeAsGain=off  AntiWindupMode=none  Kb=1  TrackingMode=off  Kt=1  PParamMin=[]  PParamMax=[]  IParamMin=[]  IParamMax=[]  DParamMin=[]  DParamMax=[]  NParamMin=[]  NParamMax=[]  KbParamMin=[]  KbParamMax=[]  KtParamMin=[]  KtParamMax=[]  POutMin=[]  POutMax=[]  IOutMin=[]  IOutMax=[]  DOutMin=[]  DOutMax=[]  NOutMin=[]  NOutMax=[]  KbOutMin=[]  KbOutMax=[]  KtOutMin=[]  KtOutMax=[]  IntegratorOutMin=[]  IntegratorOutMax=[]  FilterOutMin=[]  FilterOutMax=[]  SumOutMin=[]  SumOutMax=[]  SumI1OutMin=[]  SumI1OutMax=[]  SumI2OutMin=[]  SumI2OutMax=[]  SumI3OutMin=[]  SumI3OutMax=[]  SumDOutMin=[]  SumDOutMax=[]  SaturationOutMin=[]  SaturationOutMax=[]  IntegratorContinuousStateAttributes=''  IntegratorStateMustResolveToSignalObject=off  IntegratorRTWStateStorageClass=Auto  FilterContinuousStateAttributes=''  FilterStateMustResolveToSignalObject=off  FilterRTWStateStorageClass=Auto  DifferentiatorICPrevScaledInput=0  DifferentiatorOutMin=[]  DifferentiatorOutMax=[]
  roll_setpoint : Outport
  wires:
  y_pos/1 -> Discrete D Controller/1
  y_error/1 -> Discrete PI Controller/1
  Discrete PI Controller/1 -> Add/1
  Discrete D Controller/1 -> Add/2
  Add/1 -> roll_setpoint/1

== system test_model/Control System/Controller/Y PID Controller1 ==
  y_error : Inport
  y_pos : Inport  Port=2
  Add : Sum  Inputs=+-
  Discrete D Controller : Derivative/Discrete D Controller  Kd=Kd  a=a
  Discrete PI Controller : simulink/Continuous/PID Controller  Controller=PI  TimeDomain=Discrete-time  SampleTime=Ts  IntegratorMethod=Forward Euler  FilterMethod=Forward Euler  Form=Parallel  UseFilter=on  ControllerParametersSource=internal  P=Kp  I=Ki  D=0  N=100  InitialConditionSource=internal  InitialConditionForIntegrator=0  InitialConditionForFilter=0  ExternalReset=none  LimitOutput=off  UpperSaturationLimit=inf  LowerSaturationLimit=-inf  LinearizeAsGain=off  AntiWindupMode=none  Kb=1  TrackingMode=off  Kt=1  PParamMin=[]  PParamMax=[]  IParamMin=[]  IParamMax=[]  DParamMin=[]  DParamMax=[]  NParamMin=[]  NParamMax=[]  KbParamMin=[]  KbParamMax=[]  KtParamMin=[]  KtParamMax=[]  POutMin=[]  POutMax=[]  IOutMin=[]  IOutMax=[]  DOutMin=[]  DOutMax=[]  NOutMin=[]  NOutMax=[]  KbOutMin=[]  KbOutMax=[]  KtOutMin=[]  KtOutMax=[]  IntegratorOutMin=[]  IntegratorOutMax=[]  FilterOutMin=[]  FilterOutMax=[]  SumOutMin=[]  SumOutMax=[]  SumI1OutMin=[]  SumI1OutMax=[]  SumI2OutMin=[]  SumI2OutMax=[]  SumI3OutMin=[]  SumI3OutMax=[]  SumDOutMin=[]  SumDOutMax=[]  SaturationOutMin=[]  SaturationOutMax=[]  IntegratorContinuousStateAttributes=''  IntegratorStateMustResolveToSignalObject=off  IntegratorRTWStateStorageClass=Auto  FilterContinuousStateAttributes=''  FilterStateMustResolveToSignalObject=off  FilterRTWStateStorageClass=Auto  DifferentiatorICPrevScaledInput=0  DifferentiatorOutMin=[]  DifferentiatorOutMax=[]
  y_vel_setpoint : Outport
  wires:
  y_pos/1 -> Discrete D Controller/1
  y_error/1 -> Discrete PI Controller/1
  Discrete PI Controller/1 -> Add/1
  Discrete D Controller/1 -> Add/2
  Add/1 -> y_vel_setpoint/1

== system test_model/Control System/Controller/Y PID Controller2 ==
  x_error : Inport
  x_pos : Inport  Port=2
  Add : Sum  Inputs=+-
  Discrete D Controller : Derivative/Discrete D Controller  Kd=Kd  a=a
  Discrete PI Controller : simulink/Continuous/PID Controller  Controller=PI  TimeDomain=Discrete-time  SampleTime=Ts  IntegratorMethod=Forward Euler  FilterMethod=Forward Euler  Form=Parallel  UseFilter=on  ControllerParametersSource=internal  P=Kp  I=Ki  D=0  N=100  InitialConditionSource=internal  InitialConditionForIntegrator=0  InitialConditionForFilter=0  ExternalReset=none  LimitOutput=off  UpperSaturationLimit=inf  LowerSaturationLimit=-inf  LinearizeAsGain=off  AntiWindupMode=none  Kb=1  TrackingMode=off  Kt=1  PParamMin=[]  PParamMax=[]  IParamMin=[]  IParamMax=[]  DParamMin=[]  DParamMax=[]  NParamMin=[]  NParamMax=[]  KbParamMin=[]  KbParamMax=[]  KtParamMin=[]  KtParamMax=[]  POutMin=[]  POutMax=[]  IOutMin=[]  IOutMax=[]  DOutMin=[]  DOutMax=[]  NOutMin=[]  NOutMax=[]  KbOutMin=[]  KbOutMax=[]  KtOutMin=[]  KtOutMax=[]  IntegratorOutMin=[]  IntegratorOutMax=[]  FilterOutMin=[]  FilterOutMax=[]  SumOutMin=[]  SumOutMax=[]  SumI1OutMin=[]  SumI1OutMax=[]  SumI2OutMin=[]  SumI2OutMax=[]  SumI3OutMin=[]  SumI3OutMax=[]  SumDOutMin=[]  SumDOutMax=[]  SaturationOutMin=[]  SaturationOutMax=[]  IntegratorContinuousStateAttributes=''  IntegratorStateMustResolveToSignalObject=off  IntegratorRTWStateStorageClass=Auto  FilterContinuousStateAttributes=''  FilterStateMustResolveToSignalObject=off  FilterRTWStateStorageClass=Auto  DifferentiatorICPrevScaledInput=0  DifferentiatorOutMin=[]  DifferentiatorOutMax=[]
  x_vel_setpoint : Outport
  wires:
  x_pos/1 -> Discrete D Controller/1
  x_error/1 -> Discrete PI Controller/1
  Discrete PI Controller/1 -> Add/1
  Discrete D Controller/1 -> Add/2
  Add/1 -> x_vel_setpoint/1

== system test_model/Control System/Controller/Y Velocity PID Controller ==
  y_error : Inport
  y_pos : Inport  Port=2
  Add : Sum  Inputs=+-
  Discrete D Controller : Derivative/Discrete D Controller  Kd=Kd  a=a
  Discrete PI Controller : simulink/Continuous/PID Controller  Controller=PI  TimeDomain=Discrete-time  SampleTime=Ts  IntegratorMethod=Forward Euler  FilterMethod=Forward Euler  Form=Parallel  UseFilter=on  ControllerParametersSource=internal  P=Kp  I=Ki  D=0  N=100  InitialConditionSource=internal  InitialConditionForIntegrator=0  InitialConditionForFilter=0  ExternalReset=none  LimitOutput=off  UpperSaturationLimit=inf  LowerSaturationLimit=-inf  LinearizeAsGain=off  AntiWindupMode=none  Kb=1  TrackingMode=off  Kt=1  PParamMin=[]  PParamMax=[]  IParamMin=[]  IParamMax=[]  DParamMin=[]  DParamMax=[]  NParamMin=[]  NParamMax=[]  KbParamMin=[]  KbParamMax=[]  KtParamMin=[]  KtParamMax=[]  POutMin=[]  POutMax=[]  IOutMin=[]  IOutMax=[]  DOutMin=[]  DOutMax=[]  NOutMin=[]  NOutMax=[]  KbOutMin=[]  KbOutMax=[]  KtOutMin=[]  KtOutMax=[]  IntegratorOutMin=[]  IntegratorOutMax=[]  FilterOutMin=[]  FilterOutMax=[]  SumOutMin=[]  SumOutMax=[]  SumI1OutMin=[]  SumI1OutMax=[]  SumI2OutMin=[]  SumI2OutMax=[]  SumI3OutMin=[]  SumI3OutMax=[]  SumDOutMin=[]  SumDOutMax=[]  SaturationOutMin=[]  SaturationOutMax=[]  IntegratorContinuousStateAttributes=''  IntegratorStateMustResolveToSignalObject=off  IntegratorRTWStateStorageClass=Auto  FilterContinuousStateAttributes=''  FilterStateMustResolveToSignalObject=off  FilterRTWStateStorageClass=Auto  DifferentiatorICPrevScaledInput=0  DifferentiatorOutMin=[]  DifferentiatorOutMax=[]
  roll_setpoint : Outport
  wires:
  y_pos/1 -> Discrete D Controller/1
  y_error/1 -> Discrete PI Controller/1
  Discrete PI Controller/1 -> Add/1
  Discrete D Controller/1 -> Add/2
  Add/1 -> roll_setpoint/1

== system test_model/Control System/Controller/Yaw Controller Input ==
  note: 1) Add Subsystem or Model blocks as valid variant choices. 2) You cannot connect blocks at this level. At simulation, connectivity is automatically determined, based on the active variant and port name matching.
  yaw_error_model : Inport
  yaw_angle_model : Inport  Port=2
  Feedback : Subsystem  VariantControl=logAnalysisToggle==0
  yaw error : Subsystem  VariantControl=logAnalysisToggle==1
  yaw_error : Outport
  yaw_angle : Outport  Port=2

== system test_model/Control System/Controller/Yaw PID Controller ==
  yaw_error : Inport
  yaw_angle : Inport  Port=2
  Add : Sum  Inputs=+-
  Discrete D Controller : Derivative/Discrete D Controller  Kd=Kd  a=a
  Discrete PI Controller : simulink/Continuous/PID Controller  Controller=PI  TimeDomain=Discrete-time  SampleTime=Ts  IntegratorMethod=Forward Euler  FilterMethod=Forward Euler  Form=Parallel  UseFilter=on  ControllerParametersSource=internal  P=Kp  I=Ki  D=0  N=100  InitialConditionSource=internal  InitialConditionForIntegrator=0  InitialConditionForFilter=0  ExternalReset=none  LimitOutput=off  UpperSaturationLimit=inf  LowerSaturationLimit=-inf  LinearizeAsGain=off  AntiWindupMode=none  Kb=1  TrackingMode=off  Kt=1  PParamMin=[]  PParamMax=[]  IParamMin=[]  IParamMax=[]  DParamMin=[]  DParamMax=[]  NParamMin=[]  NParamMax=[]  KbParamMin=[]  KbParamMax=[]  KtParamMin=[]  KtParamMax=[]  POutMin=[]  POutMax=[]  IOutMin=[]  IOutMax=[]  DOutMin=[]  DOutMax=[]  NOutMin=[]  NOutMax=[]  KbOutMin=[]  KbOutMax=[]  KtOutMin=[]  KtOutMax=[]  IntegratorOutMin=[]  IntegratorOutMax=[]  FilterOutMin=[]  FilterOutMax=[]  SumOutMin=[]  SumOutMax=[]  SumI1OutMin=[]  SumI1OutMax=[]  SumI2OutMin=[]  SumI2OutMax=[]  SumI3OutMin=[]  SumI3OutMax=[]  SumDOutMin=[]  SumDOutMax=[]  SaturationOutMin=[]  SaturationOutMax=[]  IntegratorContinuousStateAttributes=''  IntegratorStateMustResolveToSignalObject=off  IntegratorRTWStateStorageClass=Auto  FilterContinuousStateAttributes=''  FilterStateMustResolveToSignalObject=off  FilterRTWStateStorageClass=Auto  DifferentiatorICPrevScaledInput=0  DifferentiatorOutMin=[]  DifferentiatorOutMax=[]
  yawrate_setpoint : Outport
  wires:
  yaw_angle/1 -> Discrete D Controller/1
  yaw_error/1 -> Discrete PI Controller/1
  Discrete PI Controller/1 -> Add/1
  Discrete D Controller/1 -> Add/2
  Add/1 -> yawrate_setpoint/1
